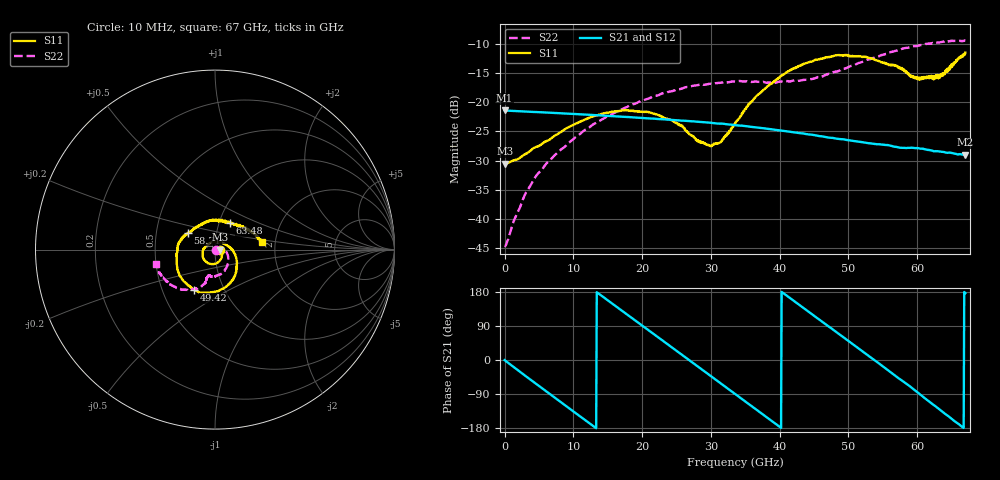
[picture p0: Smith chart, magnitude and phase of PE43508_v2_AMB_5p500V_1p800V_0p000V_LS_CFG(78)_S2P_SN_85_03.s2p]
!Keysight Technologies,N5227A,US51270237,A.10.43.00
!Date: Wednesday, August 22, 2018 17:14:46
!Correction: S11(Full 2 Port(1,3))
!S31(Full 2 Port(1,3))
!S13(Full 2 Port(1,3))
!S33(Full 2 Port(1,3))
!S2P File: Measurements: S11, S31, S13, S33:
# Hz S  dB  R 50
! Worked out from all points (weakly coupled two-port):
!   801 points, 10 MHz to 67 GHz, reference 50 ohm
!   highest |S21| = -21.40 dB at 10 MHz (marker M1); lowest = -29.0 dB at 67 GHz (marker M2)
!   lowest |S11| = -30.5 dB at 93.74 MHz (marker M3), VSWR 1.06, Z = 53.1 - j0.024 ohm
!   |S11| at or under -10 dB: start of sweep to end of sweep
!   |S22| runs from -44.7 to -9.4 dB; largest |S21 - S12| = 0.00047
!   S11 on the Smith chart (normalised r, x): 10 MHz: 1.06, -0.00; 49.42 GHz: 0.72, -0.35; 58.71 GHz: 0.73, +0.14; 63.48 GHz: 1.13, +0.34; 67 GHz: 1.71, +0.15
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1e7  -30.45 -0.8  -21.40 -0.2  -21.41 -0.2  -44.61 -1.4
9.37375e7  -30.51 -0.4  -21.42 -1.4  -21.43 -1.4  -44.67 4.3
2.857075e9  -28.97 -12.4  -21.59 -39.5  -21.59 -39.5  -36.10 35.8
4.531825e9  -27.69 -21.4  -21.68 -62.2  -21.68 -62.1  -32.74 31.3
7.3789e9  -25.66 -41.8  -21.85 -100.5  -21.85 -100.5  -28.99 19.4
1.123082e10  -23.18 -70.1  -22.08 -152.1  -22.09 -152.1  -25.18 -2.7
1.74274e10  -21.38 -114.9  -22.50 125.3  -22.50 125.3  -20.99 -33.4
2.236791e10  -22.19 -152.4  -22.88 59.4  -22.87 59.4  -18.78 -55.1
2.982055e10  -27.49 103.7  -23.49 -40.1  -23.49 -40.1  -16.84 -82.7
3.132782e10  -26.90 68.2  -23.67 -60.0  -23.67 -60.0  -16.65 -87.6
3.3505e10  -23.74 26.2  -23.92 -89.5  -23.93 -89.6  -16.43 -94.1
3.55147e10  -20.42 -0.9  -24.17 -116.5  -24.17 -116.4  -16.44 -97.9
3.836178e10  -17.19 -28.6  -24.57 -154.4  -24.58 -154.3  -16.65 -102.9
4.137632e10  -14.65 -54.2  -25.03 165.1  -25.03 165.3  -16.45 -104.5
4.472582e10  -13.00 -81.1  -25.57 120.5  -25.56 120.5  -16.02 -105.2
4.941512e10  -11.91 -117.6  -26.38 57.9  -26.38 57.9  -14.22 -106.4
5.251341e10  -12.26 -143.7  -26.93 16.3  -26.91 16.2  -12.81 -112.3
5.586291e10  -13.65 -178.2  -27.38 -29.0  -27.35 -29.4  -11.50 -122.3
5.870999e10  -15.03 147.7  -27.82 -66.4  -27.83 -66.7  -10.65 -131.9
6.130585e10  -15.88 102.3  -28.09 -103.7  -28.11 -104.1  -10.01 -142.2
6.348302e10  -15.47 60.2  -28.48 -133.8  -28.52 -134.5  -9.67 -151.3
6.7e10  -11.50 8.9  -28.99 176.7  -29.08 176.6  -9.44 -166.2
